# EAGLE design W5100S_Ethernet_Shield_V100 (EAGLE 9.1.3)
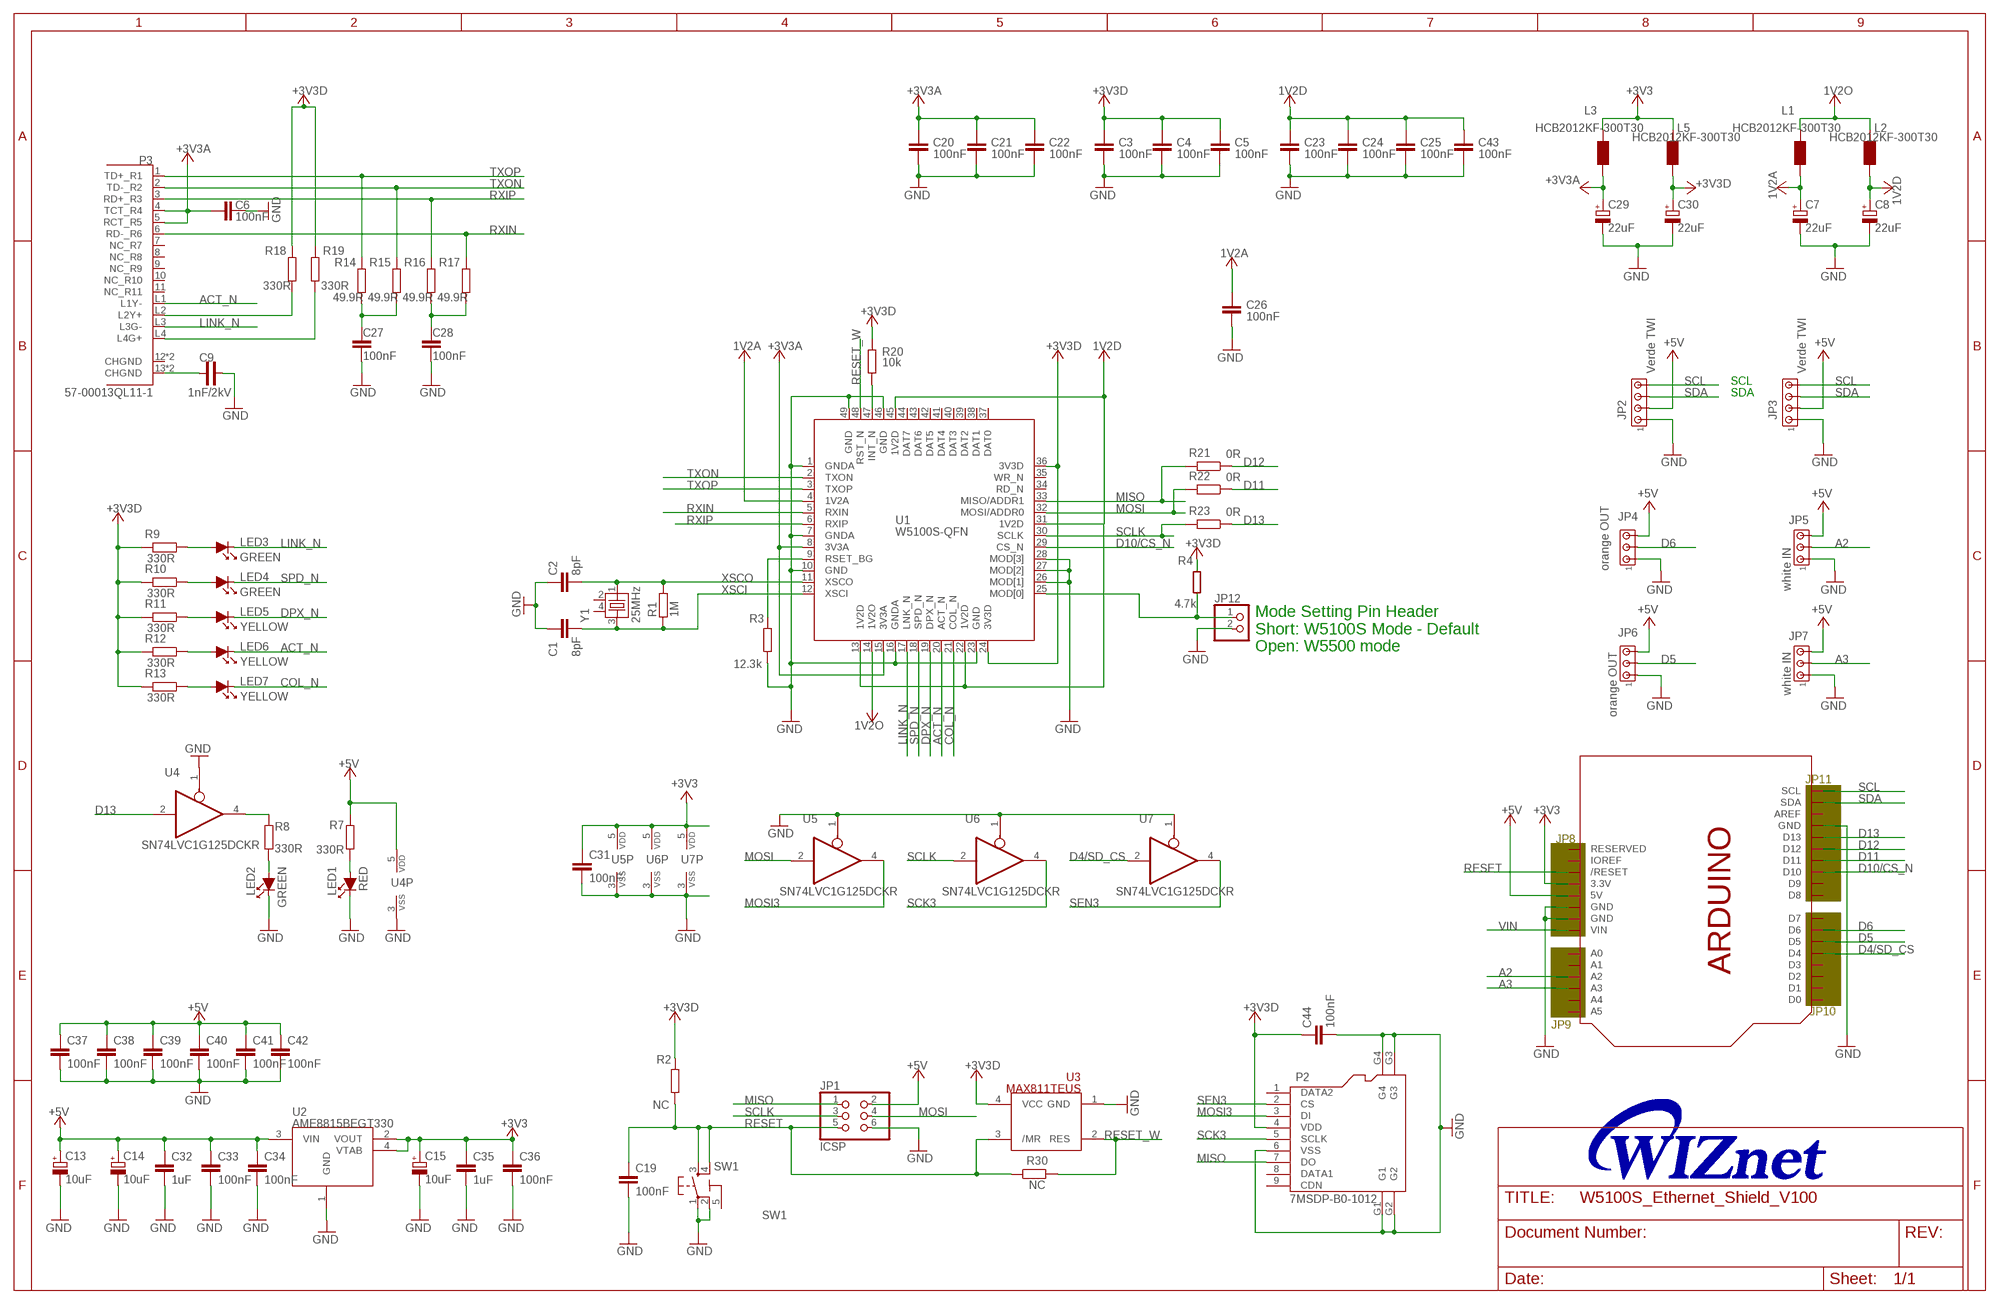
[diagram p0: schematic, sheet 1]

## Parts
C1  8pF  C-EU0603-RND  [C0603-ROUND]
C2  8pF  C-EU0603-RND  [C0603-ROUND]
C3  100nF  C-EU0603-RND  [C0603-ROUND]
C4  100nF  C-EU0603-RND  [C0603-ROUND]
C5  100nF  C-EU0603-RND  [C0603-ROUND]
C6  100nF  0142_10NF_0603  [C0603-ROUND@1]
C7  22uF  0474_TAJA475M016RNJ  [SMC_A]
C8  22uF  0474_TAJA475M016RNJ  [SMC_A]
C9  1nF/2kV  C-4520  [C-4520]
C13  10uF  0474_TAJA475M016RNJ  [SMC_A]
C14  10uF  0474_TAJA475M016RNJ  [SMC_A]
C15  10uF  0474_TAJA475M016RNJ  [SMC_A]
C19  100nF  0142_10NF_0603  [C0603-ROUND@1]
C20  100nF  C-EU0603-RND  [C0603-ROUND]
C21  100nF  C-EU0603-RND  [C0603-ROUND]
C22  100nF  C-EU0603-RND  [C0603-ROUND]
C23  100nF  C-EU0603-RND  [C0603-ROUND]
C24  100nF  C-EU0603-RND  [C0603-ROUND]
C25  100nF  C-EU0603-RND  [C0603-ROUND]
C26  100nF  C-EU0603-RND  [C0603-ROUND]
C27  100nF  0142_10NF_0603  [C0603-ROUND@1]
C28  100nF  0142_10NF_0603  [C0603-ROUND@1]
C29  22uF  0474_TAJA475M016RNJ  [SMC_A]
C30  22uF  0474_TAJA475M016RNJ  [SMC_A]
C31  100nF  0006_1UF_0603/GRM188R61E105KA12D  [C0603-ROUND]
C32  1uF  0142_10NF_0603  [C0603-ROUND@1]
C33  100nF  0142_10NF_0603  [C0603-ROUND@1]
C34  100nF  0142_10NF_0603  [C0603-ROUND@1]
C35  1uF  0142_10NF_0603  [C0603-ROUND@1]
C36  100nF  0142_10NF_0603  [C0603-ROUND@1]
C37  100nF  0142_10NF_0603  [C0603-ROUND@1]
C38  100nF  0142_10NF_0603  [C0603-ROUND@1]
C39  100nF  0142_10NF_0603  [C0603-ROUND@1]
C40  100nF  0142_10NF_0603  [C0603-ROUND@1]
C41  100nF  0142_10NF_0603  [C0603-ROUND@1]
C42  100nF  0142_10NF_0603  [C0603-ROUND@1]
C43  100nF  C-EU0603-RND  [C0603-ROUND]
C44  100nF  0006_1UF_0603/GRM188R61E105KA12D  [C0603-ROUND]
JP1  ICSP  0114_PH254-203DF118A00V  [2X03]
JP2  Verde TWI  1693_WA254-04S-632  [10X04MTA]
JP3  Verde TWI  1693_WA254-04S-632  [10X04MTA]
JP4  orange OUT  1696_WA254-03S-166  [10X03MTA]
JP5  white IN  1695_WA254-03S-IN  [10X03MTA]
JP6  orange OUT  0141_LHA-03-TS  [10X03MTA]
JP7  white IN  1695_WA254-03S-IN  [10X03MTA]
JP12  PINHD-1X2  [1X02]
L1  HCB2012KF-300T30  0001_BLM21PG300SN1D_/_MH2029-300Y  [0805]
L2  HCB2012KF-300T30  0001_BLM21PG300SN1D_/_MH2029-300Y  [0805]
L3  HCB2012KF-300T30  0001_BLM21PG300SN1D_/_MH2029-300Y  [0805]
L5  HCB2012KF-300T30  0001_BLM21PG300SN1D_/_MH2029-300Y  [0805]
LED1  RED  LED-1608  [LED-1608]
LED2  GREEN  LED-1608  [LED-1608]
LED3  GREEN  LED-1608  [LED-1608]
LED4  GREEN  LED-1608  [LED-1608]
LED5  YELLOW  LED-1608  [LED-1608]
LED6  YELLOW  LED-1608  [LED-1608]
LED7  YELLOW  LED-1608  [LED-1608]
P2  7MSDP-B0-1012  MICRO-SD-CARD-SOCKET-9P(ST-TF-003A)  [MICRO-SD9+4P-SMD-16.1X14.5X1.85MM]
P3  57-00013QL11-1  [57-00013QL11-1]
R1  1M  RESISTENZE_0026_100K_0603  [RESISTENZE_R0603-ROUND]
R2  NC  0028_CR0603JW103L  [R0603-ROUND]
R3  12.3k  0028_CR0603JW103L  [R0603-ROUND]
R4  4.7k  R-330R-0402  [0402-1005X55N]
R7  330R  RESISTENZE_0026_100K_0603  [RESISTENZE_R0603-ROUND]
R8  330R  RESISTENZE_0026_100K_0603  [RESISTENZE_R0603-ROUND]
R9  330R  0028_CR0603JW103L  [R0603-ROUND]
R10  330R  0028_CR0603JW103L  [R0603-ROUND]
R11  330R  0028_CR0603JW103L  [R0603-ROUND]
R12  330R  0028_CR0603JW103L  [R0603-ROUND]
R13  330R  0028_CR0603JW103L  [R0603-ROUND]
R14  49.9R  RESISTENZE_0026_100K_0603  [RESISTENZE_R0603-ROUND]
R15  49.9R  RESISTENZE_0026_100K_0603  [RESISTENZE_R0603-ROUND]
R16  49.9R  RESISTENZE_0026_100K_0603  [RESISTENZE_R0603-ROUND]
R17  49.9R  RESISTENZE_0026_100K_0603  [RESISTENZE_R0603-ROUND]
R18  330R  RESISTENZE_0026_100K_0603  [RESISTENZE_R0603-ROUND]
R19  330R  RESISTENZE_0026_100K_0603  [RESISTENZE_R0603-ROUND]
R20  10k  0028_CR0603JW103L  [R0603-ROUND]
R21  0R  0028_CR0603JW103L  [R0603-ROUND]
R22  0R  0028_CR0603JW103L  [R0603-ROUND]
R23  0R  0028_CR0603JW103L  [R0603-ROUND]
R30  NC  0028_CR0603JW103L  [R0603-ROUND]
SW1  SW1  0946_TS42031-160W-TR-7260  [TS42]
U1  W5100S-QFN  [W5100S-QFN]
U2  AME8815BEGT330  [SOT-223]
U3  MAX811TEUS  0035_CAT811TTBI-GT3  [SOT143]
U4  SN74LVC1G125DCKR  0040_SN74LVC1G125DCKR  [SC70-5]
U5  SN74LVC1G125DCKR  0040_SN74LVC1G125DCKR  [SC70-5]
U6  SN74LVC1G125DCKR  0040_SN74LVC1G125DCKR  [SC70-5]
U7  SN74LVC1G125DCKR  0040_SN74LVC1G125DCKR  [SC70-5]
U$4  ARDUINO_R3_ICSP_4  [ARDUINOR3_ICSP_4]
Y1  25MHz  XTAL3225  [XTAL3225]

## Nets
1V2A: C7.+ C26.2 L1.1 U1.4(1V2A)
1V2D: C8.+ C23.2 C24.2 C25.2 C43.2 L2.1 U1.13(1V2D) U1.22(1V2D) U1.31(1V2D) U1.45(1V2D)
1V2O: L1.2 L2.2 U1.14(1V2O)
+3V3 [power]: C15.+ C31.1 C35.1 C36.1 L3.2 L5.2 U2.2(VOUT) U2.4(VTAB) U5.5(VDD) U6.5(VDD) U7.5(VDD) U$4.3V(3.3V)
+3V3A [power]: C6.1 C20.2 C21.2 C22.2 C29.+ L3.1 P3.4(TCT_R4) P3.5(RCT_R5) U1.8(3V3A) U1.15(3V3A)
+3V3D: C3.2 C4.2 C5.2 C30.+ C44.1 L5.1 P2.4(VDD) R2.2 R4.2 R9.2 R10.2 R11.2 R12.2 R13.2 R18.1 R19.1 R20.2 U1.24(3V3D) U1.36(3V3D) U3.4(VCC)
+5V [power]: C13.+ C14.+ C32.1 C33.1 C34.1 C37.1 C38.1 C39.1 C40.1 C41.1 C42.1 JP1.2 JP2.2 JP3.2 JP4.3 JP5.3 JP6.3 JP7.3 R7.2 U2.3(VIN) U4.5(VDD) U$4.5V
A2: JP5.2 U$4.A2
A3: JP7.2 U$4.A3
ACT_N: LED6.K P3.L1(L1Y-) U1.20(ACT_N)
COL_N: LED7.K U1.21(COL_N)
D4/SD_CS: U7.2(I) U$4.D4
D5: JP6.2 U$4.D5
D6: JP4.2 U$4.D6
D10/CS_N: U1.29(CS_N) U$4.D10
D11: R22.1 U$4.D11
D12: R21.1 U$4.D12
D13: R23.1 U4.2(I) U$4.D13
DPX_N: LED5.K U1.19(DPX_N)
GND [gnd]: C1.1 C2.1 C3.1 C4.1 C5.1 C6.2 C7.- C8.- C9.2 C13.- C14.- C15.- C19.2 C20.1 C21.1 C22.1 C23.1 C24.1 C25.1 C26.1 C27.1 C28.1 C29.- C30.- C31.2 C32.2 C33.2 C34.2 C35.2 C36.2 C37.2 C38.2 C39.2 C40.2 C41.2 C42.2 C43.1 C44.2 JP1.6 JP2.1 JP3.1 JP4.1 JP5.1 JP6.1 JP7.1 JP12.2 LED1.K LED2.K P2.6(VSS) P2.G1 P2.G2 P2.G3 P2.G4 R3.1 SW1.1 SW1.2 U1.1(GNDA) U1.7(GNDA) U1.10(GND) U1.16(GNDA) U1.23(GND) U1.26(MOD[1]) U1.27(MOD[2]) U1.28(MOD[3]) U1.46(GND) U1.49(GND) U2.1(GND) U3.1(GND) U4.1(OE) U4.3(VSS) U5.1(OE) U5.3(VSS) U6.1(OE) U6.3(VSS) U7.1(OE) U7.3(VSS) U$4.GND U$4.GND@1(GND) U$4.GND@2(GND)
LINK_N: LED3.K P3.L3(L3G-) U1.17(LNK_N)
MISO: JP1.1 P2.7(DO) R21.2 U1.33(MISO/ADDR1)
MOSI: JP1.4 R22.2 U1.32(MOSI/ADDR0) U5.2(I)
MOSI3: P2.3(DI) U5.4(O)
N$1: LED3.A R9.1
N$2: P3.L2(L2Y+) R18.2
N$3: LED1.A R7.1
N$4: LED4.A R10.1
N$5: LED5.A R11.1
N$6: LED6.A R12.1
N$7: LED7.A R13.1
N$8: P3.L4(L4G+) R19.2
N$9: C9.1 P3.13(CHGND) P3.P$4(CHGND)
N$12: C27.2 R14.2 R15.2
N$13: R8.2 U4.4(O)
N$14: LED2.A R8.1
N$15: C28.2 R16.2 R17.2
N$16: R20.1 U1.47(INT_N)
N$17: JP12.1 R4.1 U1.25(MOD[0])
N$20: R3.2 U1.9(RSET_BG)
RESET: C19.1 JP1.5 R2.1 R30.1 SW1.3 SW1.4 U3.3(/MR) U$4.RESET(/RESET)
RESET_W: R30.2 U1.48(RST_N) U3.2(RES)
RXIN: P3.6(RD-_R6) R17.1 U1.5(RXIN)
RXIP: P3.3(RD+_R3) R16.1 U1.6(RXIP)
SCK3: P2.5(SCLK) U6.4(O)
SCL: JP2.4 JP3.4 U$4.SCL
SCLK: JP1.3 R23.2 U1.30(SCLK) U6.2(I)
SDA: JP2.3 JP3.3 U$4.SDA
SEN3: P2.2(CS) U7.4(O)
SPD_N: LED4.K U1.18(SPD_N)
TXON: P3.2(TD-_R2) R15.1 U1.2(TXON)
TXOP: P3.1(TD+_R1) R14.1 U1.3(TXOP)
VIN [gnd]: U$4.VIN
XSCI: C1.2 R1.1 U1.12(XSCI) Y1.3
XSCO: C2.2 R1.2 U1.11(XSCO) Y1.1
Unconnected: P2.1(DATA2) P2.8(DATA1) P2.9(CDN) P3.7(NC_R7) P3.8(NC_R8) P3.9(NC_R9) P3.10(NC_R10) P3.11(NC_R11) P3.12(CHGND) P3.P$3(CHGND) U1.34(RD_N) U1.35(WR_N) U1.37(DAT0) U1.38(DAT1) U1.39(DAT2) U1.40(DAT3) U1.41(DAT4) U1.42(DAT5) U1.43(DAT6) U1.44(DAT7) U$4.A0 U$4.A1 U$4.A4 U$4.A5 U$4.AREF U$4.D0 U$4.D1 U$4.D2 U$4.D3 U$4.D7 U$4.D8 U$4.D9 U$4.IOREF U$4.RESERVED Y1.2 Y1.4

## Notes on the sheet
- SCL
- SDA
- Mode Setting Pin Header
  Short: W5100S Mode - Default
  Open: W5500 mode
- JP11
- JP8
- JP10
- JP9

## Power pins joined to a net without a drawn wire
5-GND: SW1.5(5-GND)

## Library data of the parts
C1-C5 C20-C26 C43 = SmartPrj:C-EU: CAPACITOR, European symbol
C6 C19 C27 C28 C32-C42 = Condensatori:0142_10NF_0603: 10nF 0603; CASE: 0603; MONTHLY_USAGE: _____; PART_NUMBER: 10nF_0603; PRICE: _____; SUPPLIER: _____; TYPE: Condensatori; VALUE: 10nF
C7 C8 C13-C15 C29 C30 = Condensatori:0474_TAJA475M016RNJ: 4u7 tantalio Case A - testa gialla -Tantalio; CASE: CaseA_(1206); MONTHLY_USAGE: _____; PART_NUMBER: TAJA475M016RNJ; PRICE: _____; SUPPLIER: _____; TYPE: Condensatori; VALUE: 4u7
C9 = CAP:C-4520
C31 C44 = Condensatori:0006_1UF_0603/GRM188R61E105KA12D: 1uF 0603; CASE: 0603; MONTHLY_USAGE: 207014.16; PART_NUMBER: 1uF_0603/GRM188R61E105KA12D; PRICE: �_0.00; SUPPLIER: La_Tecnika_Due_s.r.l.; TYPE: Condensatori; VALUE: 1uF
JP1 = Connettori:0114_PH254-203DF118A00V: 3x2 M V h 8,5 mm p2,54; MONTHLY_USAGE: _____; PART_NUMBER: PH254-203DF118A00V; PRICE: _____; SUPPLIER: _____; TYPE: Connettori
JP2 JP3 = Connettori:1693_WA254-04S-632: 4x1 V Verde p 2,54 Serigrafato TWI; MONTHLY_USAGE: _____; PART_NUMBER: WA254-04S-632; PRICE: _____; SUPPLIER: _____; TYPE: Connettori; VALUE: WA254-04S-632
JP4 = Connettori:1696_WA254-03S-166: 3x1 Poli V Arancioni Serigrafati OUT; MONTHLY_USAGE: _____; PART_NUMBER: WA254-03S-166; PRICE: _____; SUPPLIER: _____; TYPE: Connettori; VALUE: WA254-03S-166
JP5 JP7 = Connettori:1695_WA254-03S-IN: 3x1 V Bianco P2,54 Serigrafati IN; MONTHLY_USAGE: _____; PART_NUMBER: WA254-03S-IN; PRICE: _____; SUPPLIER: _____; TYPE: Connettori; VALUE: WA254-03S-IN
JP6 = Connettori:0141_LHA-03-TS: 3x1 V Bianco P2,54; MONTHLY_USAGE: _____; PART_NUMBER: LHA-03-TS; PRICE: _____; SUPPLIER: _____; TYPE: Connettori; VALUE: LHA-03-TS
JP12 = PinHeader:PINHD-1X2: PIN HEADER
L1-L3 L5 = Protezione:0001_BLM21PG300SN1D_/_MH2029-300Y: BLM21; MONTHLY_USAGE: _____; PART_NUMBER: BLM21PG300SN1D_/_MH2029-300Y; PRICE: _____; SUPPLIER: _____; TYPE: Protezione; VALUE: MH2029-300Y
LED1-LED7 = DIODE:LED-1608
P2 = Seeed-OPL-Connector:MICRO-SD-CARD-SOCKET-9P(ST-TF-003A): 320090000; MPN: ST-TF-003A; VALUE: ST-TF-003A
P3 = WIZnet:57-00013QL11-1
R1 R7 R8 R14-R19 = Arduino-M0-V1:RESISTENZE_0026_100K_0603: 100K 0603; CASE: 0603; MONTHLY_USAGE: _____; PART_NUMBER: 100K_0603; PRICE: _____; SUPPLIER: _____; TYPE: Resistenze; VALUE: 100k
R2 R3 R9-R13 R21-R23 R30 = Resistenze:0028_CR0603JW103L: 10K 0603; CASE: 0603; MONTHLY_USAGE: _____; PART_NUMBER: CR0603JW103L; PRICE: _____; SUPPLIER: _____; TYPE: Resistenze; VALUE: 10k
R4 = MK1_Zero:R: Resistor; DESCR: RES 330 OHM 1/16W 1% 0402 SMD; MF: Yageo; MPN: RC0402FR-07330RL
R20 = Resistenze:0028_CR0603JW103L: 10K 0603; CASE: 0603; MONTHLY_USAGE: _____; PART_NUMBER: CR0603JW103L; PRICE: _____; SUPPLIER: _____; TYPE: Resistenze
SW1 = Switches:0946_TS42031-160W-TR-7260: Pushbutton 6x6 Smd - White; MONTHLY_USAGE: _____; PART_NUMBER: IT-1157AHNP-160G-G_GTR; PRICE: _____; SUPPLIER: _____; TYPE: Switches; VALUE: TS42
U1 = WIZnet:W5100S-QFN
U2 = RECULATOR:AME8815BEGT330
U3 = Circuito Integrato:0035_CAT811TTBI-GT3: 4-Pin Microprocessor Power Supply Supervisors- Reset Controller CAT811TTBI-GT3; CASE: SOT143-4; MONTHLY_USAGE: _____; PART_NUMBER: CAT811TTBI-GT3; PRICE: _____; SUPPLIER: _____; TYPE: Circuito_Integrato; VALUE: CAT811TTBI-GT3
U4-U7 = Circuito Integrato:0040_SN74LVC1G125DCKR: Single bus buffer with 3-state output; CASE: SC70; MONTHLY_USAGE: _____; PART_NUMBER: SN74LVC1G125DCKR; PRICE: _____; SPICEPREFIX: U; SUPPLIER: _____; TYPE: Circuito_Integrato; VALUE: 74LVC1G125DCKR
U$4 = Arduino:ARDUINO_R3_ICSP_4
Y1 = X-TAL:XTAL3225

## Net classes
1 power: width 0.254 mm, drill 0.61 mm, clearance 0.203 mm
2 gnd: width 0.254 mm, drill 0.3 mm, clearance 0.127 mm

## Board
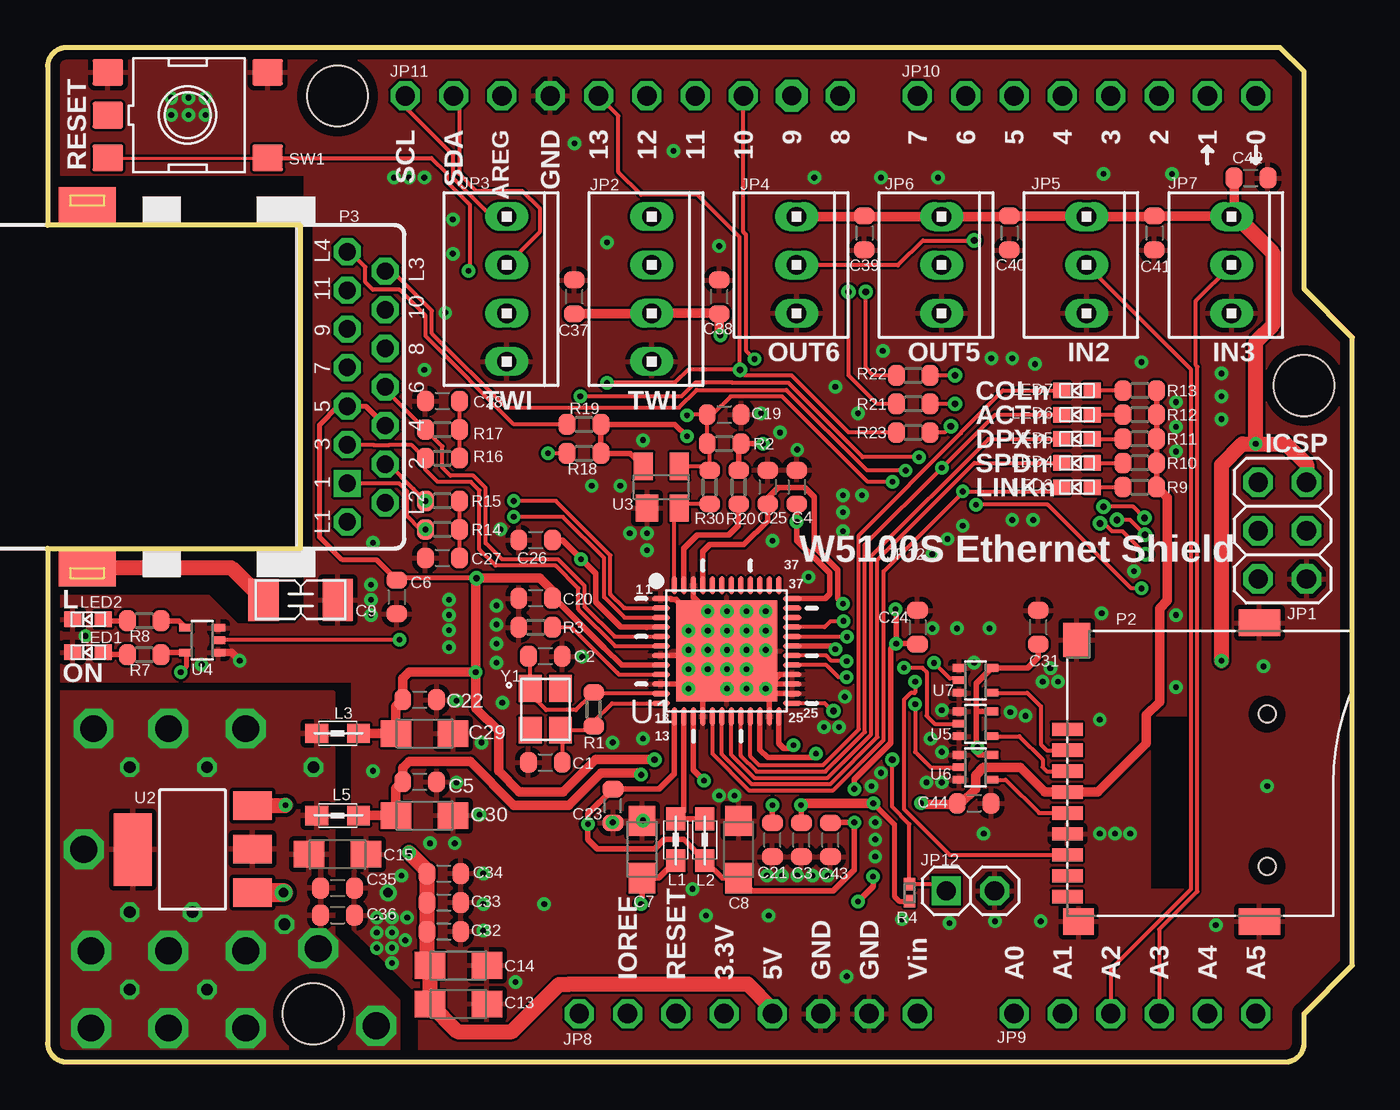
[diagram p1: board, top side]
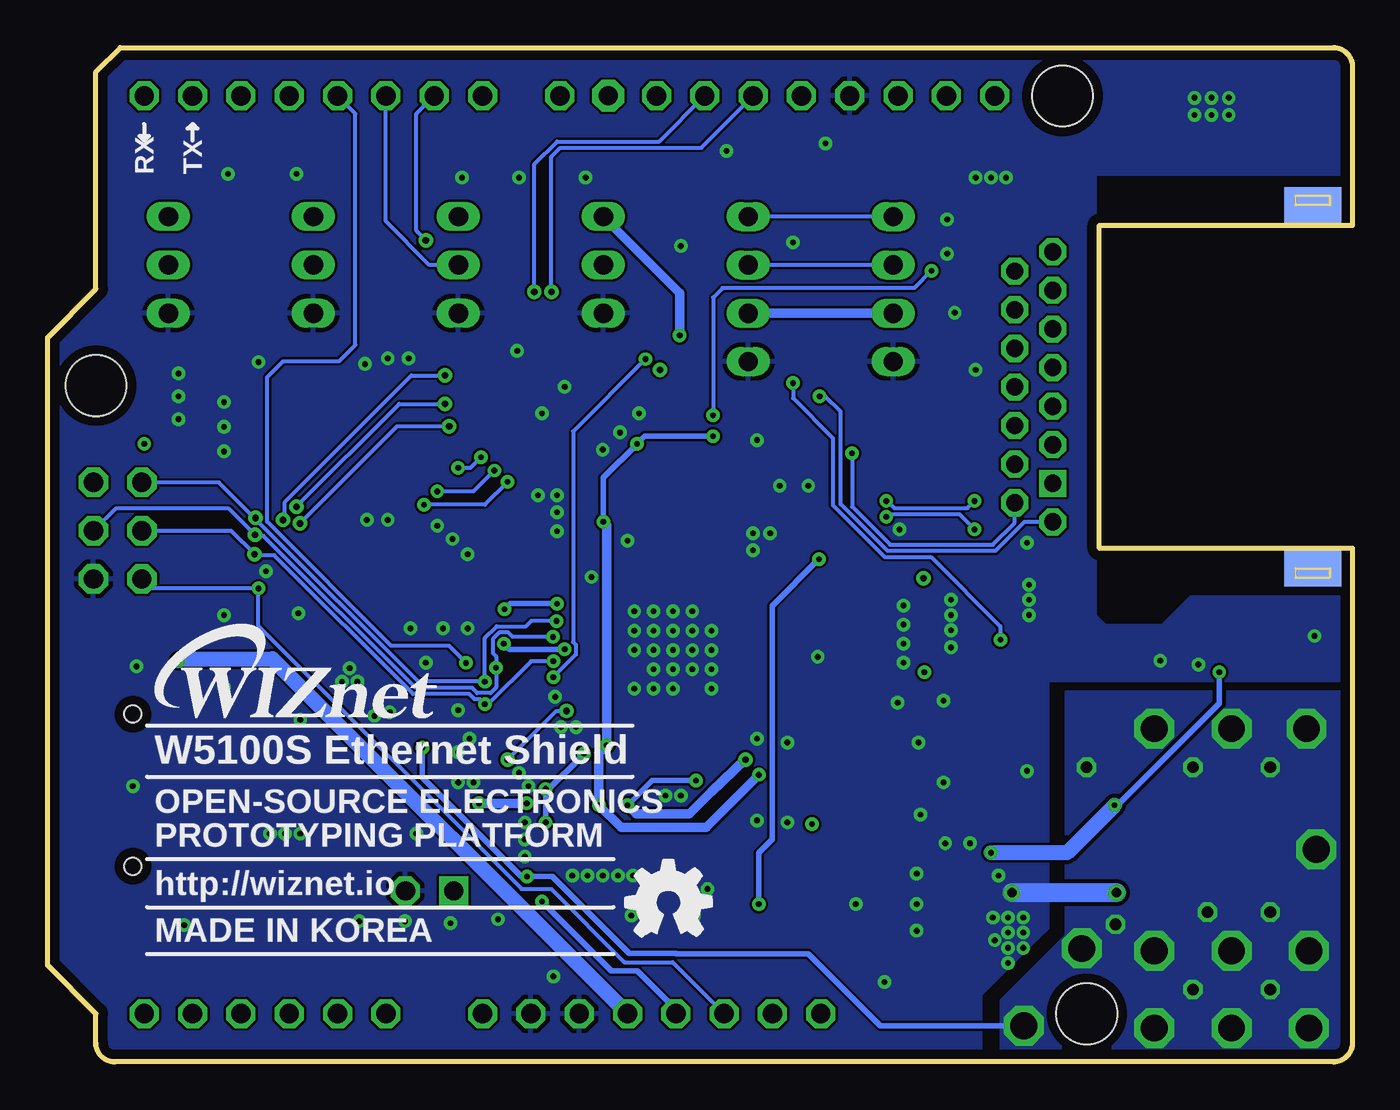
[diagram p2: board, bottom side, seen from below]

Size 68.58 x 53.34 mm. Coordinates in mm from the lower left corner, seen from the top.
Outline: 66.04,2.54 68.58,5.08 68.58,38.1 66.04,40.64 66.04,52.07 64.77,53.34 1,53.34 arc90 0,52.34 0,44 13.3,44 13.3,27 0,27 0,1 arc90 1,0 65.04,0 arc90 66.04,1 66.04,2.54
Copper layers (1*16): Top 0.035mm / dielectric 1.5mm / Bottom 0.035mm
Design rules "default *": minimum track width 6mil, minimum drill 0.2mm, track to track 5mil, track to pad 5mil, pad to pad 5mil, via to via 5mil, smd to smd 4mil, copper to edge 20mil, drill to drill 10mil, minimum pad ring 10mil, minimum via ring 8mil, stop-mask expansion 1mil, vias tented up to drill 15mil, thermal gap 10mil

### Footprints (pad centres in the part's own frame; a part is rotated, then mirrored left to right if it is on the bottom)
C0603-ROUND = smd 0.898 x 1.1: 1 -0.889,0; 2 0.889,0
C0603-ROUND@1 = smd 0.898 x 1.1: 1 -0.889,0; 2 0.889,0
SMC_A = smd 1.6 x 1.4: + -1.5,0; - 1.5,0
C-4520 = smd 1.6 x 2.2: 1 -1.95,0; 2 1.95,0
2X03 = drill 1.016 pad 1.55 octagon: 1 -2.54,-1.27; 2 -2.54,1.27; 3 0,-1.27; 4 0,1.27; 5 2.54,-1.27; 6 2.54,1.27
10X04MTA = drill 1.016 long: 1 3.81,0; 2 1.27,0; 3 -1.27,0; 4 -3.81,0
10X03MTA = drill 1.016 long: 1 2.54,0; 2 0,0; 3 -2.54,0
1X02 = drill 1.016 square: 1 -1.27,0 | drill 1.016 octagon: 2 1.27,0
0805 = smd 1.2 x 1: 1 -1.1,0; 2 1.1,0
LED-1608 = smd 0.89 x 0.82: A -0.8,0; K 0.8,0
MICRO-SD9+4P-SMD-16.1X14.5X1.85MM = smd 1.6 x 0.7: 1 0,2.25; 2 0,1.15; 3 0,0.05; 4 0,-1.05; 5 0,-2.15; 6 0,-3.25; 7 0,-4.35; 8 0,-5.45; 9 0,-6.55 | smd 1.6 x 1.4: G1 0.6,-7.85 | smd 2.2 x 1.4: G2 10.1,-7.85; G3 10.1,7.85 | smd 1.4 x 1.8: G4 0.5,6.95 | hole 0.9: 10.5,-4.95; 10.5,3.05
57-00013QL11-1 = drill 0.914 square: 1 5.075,10.15 | drill 0.914 octagon: 2 4.065,12.15; 3 3.045,10.15; 4 2.035,12.15; 5 1.015,10.15; 6 0.005,12.15; 7 -1.015,10.15; 8 -2.025,12.15; 9 -3.045,10.15; 10 -4.055,12.15; 11 -5.075,10.15; L1 7.105,10.15; L2 6.095,12.15; L3 -6.085,12.15; L4 -7.105,10.15 | smd 2 x 3: 12 -9.5,-3.51; 13 9.5,-3.51 | smd 2 x 3 bottom: P$3 -9.5,-3.51; P$4 9.5,-3.51
RESISTENZE_R0603-ROUND = smd 0.898 x 1.1: 1 -0.889,0; 2 0.889,0
R0603-ROUND = smd 0.898 x 1.1: 1 -0.889,0; 2 0.889,0
0402-1005X55N = smd 0.62 x 0.62: 1 -0.45,0; 2 0.45,0
TS42 = smd 1.6 x 1.4: 1 -4.2,2.25; 2 4.2,2.25; 3 -4.2,-2.25; 4 4.2,-2.25; 5 -4.2,0
W5100S-QFN = smd 0.95 x 0.25: 1 -3.45,2.75; 2 -3.45,2.25; 3 -3.45,1.75; 4 -3.45,1.25; 5 -3.45,0.75; 6 -3.45,0.25; 7 -3.45,-0.25; 8 -3.45,-0.75; 9 -3.45,-1.25; 10 -3.45,-1.75; 11 -3.45,-2.25; 12 -3.45,-2.75; 25 3.45,-2.75; 26 3.45,-2.25; 27 3.45,-1.75; 28 3.45,-1.25; 29 3.45,-0.75; 30 3.45,-0.25; 31 3.45,0.25; 32 3.45,0.75; 33 3.45,1.25; 34 3.45,1.75; 35 3.45,2.25; 36 3.45,2.75 | smd 0.25 x 0.95: 13 -2.75,-3.45; 14 -2.25,-3.45; 15 -1.75,-3.45; 16 -1.25,-3.45; 17 -0.75,-3.45; 18 -0.25,-3.45; 19 0.25,-3.45; 20 0.75,-3.45; 21 1.25,-3.45; 22 1.75,-3.45; 23 2.25,-3.45; 24 2.75,-3.45; 37 2.75,3.45; 38 2.25,3.45; 39 1.75,3.45; 40 1.25,3.45; 41 0.75,3.45; 42 0.25,3.45; 43 -0.25,3.45; 44 -0.75,3.45; 45 -1.25,3.45; 46 -1.75,3.45; 47 -2.25,3.45; 48 -2.75,3.45 | smd 5.3 x 5.3: 49 0,0
SOT-223 = smd 1.499 x 2.007: 1 -2.261,-3.15; 2 0.025,-3.15; 3 2.311,-3.15 | smd 3.81 x 2.007: 4 0,3.15
SOT143 = smd 1.2 x 1.44: 1 -0.75,-1.1 | smd 1 x 1.44: 2 0.95,-1.1; 3 0.95,1.1; 4 -0.95,1.1
SC70-5 = smd 0.4 x 0.7: 1 -0.65,-0.85; 2 0,-0.85; 3 0.65,-0.85; 4 0.65,0.85; 5 -0.65,0.85
ARDUINOR3_ICSP_4 = drill 1.016 octagon: 3V 35.56,2.54; 5V 38.1,2.54; A0 50.8,2.54; A1 53.34,2.54; A2 55.88,2.54; A3 58.42,2.54; A4 60.96,2.54; A5 63.5,2.54; AREF 23.876,50.8; D0 63.5,50.8; D1 60.96,50.8; D2 58.42,50.8; D3 55.88,50.8; D4 53.34,50.8; D5 50.8,50.8; D6 48.26,50.8; D7 45.72,50.8; D8 41.656,50.8; D10 36.576,50.8; D11 34.036,50.8; D12 31.496,50.8; D13 28.956,50.8; GND 26.416,50.8; GND@1 43.18,2.54; GND@2 40.64,2.54; IOREF 30.48,2.54; RESERVED 27.94,2.54; RESET 33.02,2.54; SCL 18.796,50.8; SDA 21.336,50.8; VIN 45.72,2.54 | drill 1 pad 1.676 octagon: D9 39.116,50.8 | hole 3.2: 66.04,35.56; 15.24,50.8; 13.97,2.54
XTAL3225 = smd 1.4 x 1.2: 1 -1.1,-0.8; 2 1.1,-0.8; 3 1.1,0.8; 4 -1.1,0.8

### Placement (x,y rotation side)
C1  26.16,15.75 0 top
C2  26.16,21.34 180 top
C3  39.62,11.68 90 top
C4  39.37,30.23 270 top
C5  19.56,14.73 180 top
C6  18.35,24.45 270 top
C7  31.24,11.18 90 top
C8  36.32,11.18 90 top
C9  13.3,24.3 0 top
C13  21.59,3.05 0 top
C14  21.59,5.08 0 top
C15  15.24,10.92 0 top
C19  35.56,34.04 0 top
C20  25.65,24.38 0 top
C21  38.1,11.68 90 top
C22  19.56,19.05 180 top
C23  29.72,13.46 90 top
C24  45.72,22.86 270 top
C25  37.85,30.23 270 top
C26  25.65,27.44 0 top
C27  20.75,26.5 0 top
C28  20.75,34.75 0 top
C29  19.81,17.27 0 top
C30  19.81,12.95 0 top
C31  52.07,22.86 90 top
C32  20.83,6.86 0 top
C33  20.83,8.38 0 top
C34  20.83,9.91 0 top
C35  15.24,9.14 0 top
C36  15.24,7.72 0 top
C37  27.69,40.23 90 top
C38  35.31,40.23 90 top
C39  42.93,43.59 270 top
C40  50.55,43.59 270 top
C41  58.17,43.59 270 top
C42  63.25,46.48 0 top
C43  41.15,11.68 90 top
C44  48.7,13.6 0 top
JP1  64.9,27.94 270 top
JP2  31.75,40.64 270 top
JP3  24.13,40.64 270 top
JP4  39.37,41.91 270 top
JP5  54.61,41.91 270 top
JP6  46.99,41.91 270 top
JP7  62.23,41.91 270 top
JP12  48.5,9 0 top
L1  33.02,11.68 90 top
L2  34.54,11.68 90 top
L3  15.24,17.27 180 top
L5  15.24,12.95 180 top
LED1  2.13,21.54 180 top
LED2  2.13,23.28 180 top
LED3  54.1,30.23 180 top
LED4  54.1,31.5 180 top
LED5  54.1,32.77 180 top
LED6  54.1,34.04 180 top
LED7  54.1,35.31 180 top
P2  53.59,15.24 0 top
P3  5.6,35.5 270 top
R1  28.7,18.54 90 top
R2  35.56,32.51 0 top
R3  25.65,22.86 0 top
R4  45.3,8.9 270 top
R7  5.08,21.42 0 top
R8  5.08,23.2 0 top
R9  57.4,30.23 0 top
R10  57.4,31.5 0 top
R11  57.4,32.77 0 top
R12  57.4,34.04 0 top
R13  57.4,35.31 0 top
R14  20.75,28 0 top
R15  20.75,29.5 0 top
R16  20.75,31.75 0 top
R17  20.75,33.25 0 top
R18  28.19,32 180 top
R19  28.19,33.53 180 top
R20  36.32,30.23 90 top
R21  45.5,34.6 0 top
R22  45.5,36.1 0 top
R23  45.5,33.1 0 top
R30  34.8,30.23 270 top
SW1  7.37,49.78 0 top
U1  35.69,21.62 0 top
U2  7.62,11.18 90 top
U3  32.26,30.23 0 top
U4  8.13,22.18 90 top
U5  48.77,17.78 270 top
U6  48.77,15.49 270 top
U7  48.77,20.07 270 top
U$3  [WIZNET2-LOGO]  63.85,16.91 0 bottom
U$4  0,0 0 top
U$5  [OSHP-LOGO]  39,6 0 bottom
Y1  26.16,18.54 270 top

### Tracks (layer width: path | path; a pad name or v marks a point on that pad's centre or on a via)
1V2A  (via drill 0.3)
  Top 0.3: L1.1 32.11,9.68 C7.+ 31.24,8.34 v31.2,8.3 | 31.48,22.86 31.11,22.86 | v28.04,26.44 27.94,26.54 | v28.04,26.44 28.8,25.68 28.8,24.2 30.14,22.86 31.48,22.86 | v28.04,26.44 27.04,27.44 C26.2 | 31.48,22.86 U1.4
  Bottom 0.3: v28.04,26.44 30.5,23.98 30.5,11.7 31.2,11 v31.2,8.3 31.2,8.2
1V2D  (via drill 0.3)
  Top 0.3: C8.+ 35.45,9.68 L2.1 33.43,11.7 32.4,11.7 31.9,11.2 28.9,11.2 28.4,11.7 v28.4,12.5 28.4,13.03 C23.2 32.15,14.35 32.94,15.14 U1.13 | 41.23,21.86 v41.4,21.7 41.23,21.86 | v44.6,22 45.69,22 C24.2 | v40.39,16.2 40.18,16 37.85,16 37.44,16.41 U1.22 | C43.2 41.17,12.6 v42.4,12.6 42.4,10.1 41.3,9 37,9 C8.+ | C8.+ 36.6,9.4 | v44.6,22 44.32,21.72 44.32,16.79 42.4,14.87 v42.4,14.36 | v44.6,22 44.6,23.76 v44.56,23.8 | v41.8,24.1 41.53,24.37 41.53,25.88 40.3,27.1 40.3,29.7 39.8,30.2 38.4,30.2 37.85,29.65 C25.2 37.85,28.45 36.6,27.2 34.8,27.2 34.44,26.84 U1.45 | 41.23,21.86 U1.31
  Bottom 0.3: v41.4,21.7 44.3,21.7 v44.6,22 | v40.39,16.2 42.4,14.19 | 42.4,14.19 v42.4,12.6 | v42.4,14.36 42.4,14.19 | v44.56,23.8 44.26,24.1 v41.8,24.1
1V2O
  Top 0.3: L2.2 L1.2 33.44,13.2 U1.14
+3V3  (via drill 0.3, 0.61, 1.4)
  Top 0.3: U6.5 48.96,16.14 48.8,16.3 48.8,16.46 | 48.8,16.46 48.8,18.5 | 48.8,18.5 48.8,19.9 U7.5 51.52,20.72 52.07,21.27 C31.1 | U5.5 48.87,18.43 48.8,18.5 | 48.8,16.46 v48.88,16.54 | v43.39,9.75 43.39,9.22 v42.6,8.44
  Bottom 0.254: U$4.3V 35.56,2.76
  Bottom 0.3: v48.88,16.54 48.88,14.95 43.67,9.75 v43.39,9.75 42.05,9.75 38.01,5.71 35.55,5.71 35.54,5.7 28.6,5.7 24.8,1.91 v17.27,1.91 | v42.6,8.44 38.96,4.8 37.6,4.8 35.56,2.76
  other vias: 4.32,7.87 7.62,7.87 6.35,5.84 10.41,5.84 4.32,3.81 8.38,3.81 2.29,5.84 6.35,1.78 10.41,1.78 2.29,1.78 12.45,7.24 14.22,5.97 1.91,11.18 1.91,11.18 2.41,17.53 6.35,17.53 4.32,15.49 8.38,15.49 13.97,15.49 10.41,17.53
  pour Top: 0,0 18.4,0 18.4,3.2 16.4,5.2 15,6.6 15,7 15,10.4 15,16.8 15,19.4 0,19.4
  pour Bottom: 0,-0.2 18.4,-0.2 18.4,3.2 15,6.6 15,19.4 0,19.4
+3V3A  (via drill 0.3, 0.35)
  Top 0.254: v22.54,25.44 18.45,25.44 C6.1 17.29,26.4 15.5,26.4 14.3,27.6 14.3,33.5 15.29,34.48 P3.5 16.73,34.48 P3.4
  Top 0.3: 29.26,21.78 | 29.26,21.78 30.18,20.86 U1.8 | v38.1,13.5 C21.2 | v34.5,14.8 33.94,15.36 U1.15 | C20.2 26.66,24.38 29.26,21.78
  Top 0.5: L3.1 C29.+ 18.31,18.69 C22.2 18.67,20.17 19,20.5 v22.5,20.5 | v22.5,20.5 22.5,18.6 23.7,17.4 23.7,15.3 24.8,14.2 27.1,14.2 28.81,15.91 31.53,15.91 31.54,15.9 v31.9,15.9 | v22.5,20.5 22.5,25.4 v22.54,25.44 25.87,25.44 26.54,24.77 C20.2
  Bottom 0.3: v34.5,14.8 36.8,14.8 v38.1,13.5
  Bottom 0.5: v31.9,15.9 33.7,14.2 34.86,13.04 37.64,13.04 v38.1,13.5
+3V3D  (via drill 0.3)
  Top 0.254: v43.4,13.6 44.5,12.5 44.5,8.7 44.75,8.45 R4.2
  Top 0.3: C4.2 v39.37,28.4 39.37,27.43 41.1,25.7 41.1,24.6 40.87,24.36 U1.36 | v39.6,13.5 39.6,12.6 C3.2 | R13.2 R12.2 R11.2 R10.2 R9.2 | R20.2 36.32,32.38 R2.2 37.59,32.51 v37.6,32.5 | v39.2,16.66 39.04,16.5 38.7,16.5 38.44,16.76 U1.24 | v33.6,32.9 32.97,33.53 R19.1 R18.1 30.63,32 U3.4
  Top 0.5: L5.1 C30.+ 18.31,14.38 C5.2 18.67,15.47 19,15.8 22.21,15.8 24.51,13.5 27.39,13.5 29.09,15.2 31.1,15.2 v31.2,15.1 | 39.64,13.54 v39.6,13.5 39.7,13.6 v43.4,13.6 | v45.9,13.6 45.96,13.54 47.75,13.54 C44.1 48.01,13.6 48.77,14.37 48.77,15.08 49.18,15.49 51.11,15.49 52.41,14.19 P2.4 55.19,14.19 57.74,16.74 57.74,18.24 58.44,18.94 58.44,23.86 58.84,24.26 58.84,29.68 R9.2
  Bottom 0.3: v39.37,28.4 39.37,30.73 v37.6,32.5 37.2,32.9 v33.6,32.9
  Bottom 0.5: v45.9,13.6 v43.4,13.6 | v39.37,28.4 39.2,28.23 v39.2,16.66 39.6,16.26 v39.6,13.5 38.44,12.34 33.96,12.34 v31.2,15.1
+5V  (via drill 0.3)
  Top 0.254: U4.5 7.28,20.78 v7,20.5 | U$4.5V 38.1,2.8
  Top 0.3: C14.+ | U4.5 6.08,21.53 R7.2
  Top 0.5: C34.1 | 27.66,39.37 C37.1 31.72,39.34 JP2.2 35.28,39.37 C38.1 35.31,38.25 v35.36,38.2 | C42.1 62.36,44.58 62.26,44.48 | 62.26,44.48 JP7.3 | JP4.3 42.9,44.45 C39.1 42.95,44.45 JP6.3 50.52,44.45 C40.1 54.58,44.48 JP5.3 58.14,44.45 C41.1 62.26,44.48
  Top 0.8: U2.3 12.49,13.49 v12.5,13.5 | v19,11 19.93,10.07 C34.1 | C34.1 C33.1 C32.1 19.94,5.23 C14.+ | C14.+ C13.+ 21.54,1.6 24.4,1.6 26.88,4.08 27.39,4.08 27.41,4.1 36.8,4.1 38.1,2.8 | v61.7,21.1 61.7,31.4 62.8,32.5 v63.5,32.5 | v63.5,32.5 65.1,32.5 66.17,31.43 JP1.2 | v63.5,32.5 63.5,37.88 64.41,38.78 64.41,42.53 62.36,44.58
  Bottom 0.3: v12.5,13.5 12.36,13.5 7,18.86 v7,20.5
  Bottom 0.5: JP3.2 JP2.2 | v35.36,38.2 35.36,40.44 JP4.3
  Bottom 0.8: v12.5,13.5 15,11 v19,11 | v61.7,21.1 61.4,21.2 56.76,21.2 U$4.5V
A2
  Top 0.2: JP5.2 60.1,36.42 60.1,9.11 55.88,4.88 U$4.A2
A3
  Top 0.2: JP7.2 60.35,40.03 60.35,36.63 60.43,36.55 60.43,8.97 58.42,6.96 U$4.A3
ACT_N  (via drill 0.3)
  Top 0.2: LED6.K 49.8,34.04 v47,31.24 42.96,27.2 42.96,17.35 40.88,15.27 37.27,15.27 36.44,16.1 U1.20 | v45.8,31.8 42.83,31.8 38.92,35.72 36,35.72 | v28,35 33.32,35 34.03,35.71 34.03,35.72
  Top 0.203: 36,35.72 34.03,35.72
  Bottom 0.2: v45.8,31.8 46.36,31.24 v47,31.24 | P3.L1 17.24,28.39 18.77,26.87 24.43,26.87 26.9,29.34 26.9,34.2 27.7,35 v28,35
COL_N
  Top 0.2: LED7.K 50.21,35.31 48,33.1 48,33.06 42.63,27.69 42.63,17.49 40.75,15.6 37.4,15.6 36.94,16.06 U1.21
D4/SD_CS  (via drill 0.3)
  Top 0.2: U7.2 47.82,20.16 47.42,20.16 46.6,20.98 v46.58,20.98
  Bottom 0.2: v46.58,20.98 47.5,21.9 50.54,21.9 57.05,28.41 57.05,36.01 56.2,36.85 53.25,36.85 52.4,37.7 52.4,49.86 U$4.D4
D5
  Bottom 0.2: JP6.2 48.51,41.91 50.8,44.2 U$4.D5
D6  (via drill 0.35)
  Top 0.2: v48.7,43.2 46,43.2 44.7,41.9 39.38,41.9 JP4.2
  Bottom 0.2: v48.7,43.2 49.2,43.7 49.2,49.86 U$4.D6
D10/CS_N  (via drill 0.3)
  Top 0.2: v42,20.24 41.56,20.24 40.94,20.86 U1.29 | v37.16,36.96 36.7,37.41 36.7,43.51 36.58,43.64 U$4.D10
  Bottom 0.2: v42,20.24 40.82,21.42 40.82,21.94 40.96,22.08 40.96,33.16 v37.16,36.96
D11  (via drill 0.35)
  Top 0.2: R22.1 43.4,36.1 43,36.5 v43,40.5
  Bottom 0.2: v43,40.5 43,47.2 41.8,48.4 36.44,48.4 U$4.D11
D12  (via drill 0.35)
  Top 0.2: R21.1 43.6,34.6 42.1,36.1 v42.1,40.5
  Bottom 0.2: v42.1,40.5 42.1,47.6 41.63,48.07 34.22,48.07 U$4.D12
D13  (via drill 0.3, 0.35)
  Top 0.2: U4.2 8.96,22.2 8.8,22.2 18.3,22.2 v18.5,22.2 | 36.38,36.42 36.38,36.5 | 36.38,36.5 36.38,43.38 34.16,45.6 31.2,45.6 30,46.8 30,49.76 U$4.D13 | R23.1 42.1,33.1 39.1,36.1 36.66,36.1 36.43,36.33 | 36.43,36.33 36.38,36.38 36.38,36.5 | v29.4,35.7 29.41,35.71 32.97,35.71 33.66,36.4 v36.4,36.4 36.4,36.36 36.43,36.33
  Bottom 0.2: v29.4,35.7 29.4,34.9 27.3,32.8 27.3,29.27 24.57,26.55 22.15,26.55 18.5,22.9 v18.5,22.2
DPX_N
  Top 0.2: LED5.K 49.45,32.77 43.29,26.6 43.29,17.22 41.02,14.95 37.13,14.95 35.94,16.14 U1.19
GND  (via drill 0.3, 0.5)
  Top 0.3: U1.16 34.44,20.39 v34.7,20.65 | 33.22,19.88 33.47,19.63 v33.68,19.63 33.44,19.87 U1.10 | U1.23 37.94,19.24 | 37.94,19.24 37.94,19.44 v37.75,19.63 37.85,19.74 | U1.26 38.06,19.36 37.94,19.24 | U1.28 38.48,20.36 37.85,19.74 | U1.27 37.98,19.86 37.85,19.74 | U1.46 33.94,24.46 v34.7,23.7 34.42,23.42 33.91,23.42 33.01,24.31 32.77,24.31 32.72,24.36 U1.1 | U1.7 33.38,21.36 v33.68,21.66
  Top 0.406: U4.1 9.67,21.53 v10.1,21.1
  Top 1: U2.1 12.38,8.91 v12.4,8.9
  Bottom 1: v12.4,8.9 v17.9,8.9
  other vias: 41.8,27.9 28.1,21.3 35.3,14 29.7,12.6 37.8,9.8 38.6,9.8 39.4,9.8 40.2,9.8 41,9.8 36.1,14 48.7,21 47,18.5 47,16.3 47,14.7 46.4,17 46.2,14.7 43.3,14.5 43.8,15.2 43.5,12.6 43.5,11.7 43.5,10.8 47.4,7.3 49.2,12 44.9,7.5 42,4.5 46.5,22.8 47.8,22.8 52.3,20 55.4,23.6 59.3,23.5 59.3,19.7 55.3,18 17.3,7.6 18.1,7.6 18.9,7.6 18.1,5.2 18.1,6.8 17.3,6.8 17.3,6 18.1,6 18.8,6.4 18.6,9.8 22.7,13 21.5,14.7 21.4,11.5 22.8,16.8 21.5,19 17.1,15.3 29.7,16.8 23.9,18.9 23.6,24 23.6,23 23.6,22 23.6,21 31.5,27.8 31.5,26.9 30.6,27.8 39.4,32.2 42.8,29.8 38.5,33.1 21.1,23.5 21.1,22.7 17,25.1 21.1,21.8 17,23.5 2,22.4 8.1,20.9 7.4,49.8 7.4,50.7 8.3,50.7 8.3,49.8 6.5,49.8 6.5,50.7 41.8,29.8 41.8,28.9 51.8,28.5 57.5,36.8 59.3,32.1 42.6,34.1 41.4,35.5 49.6,37 50.7,37 51.9,36.7 61.7,36.2 59.1,46.7 55.5,46.7 46.8,46.5 43.8,46.5 40.3,46.5 27.7,48.3 32.9,47.9 35.3,42.9 29.4,43.1 53.1,20 51.4,18.2 52.2,7.4 61.4,7.2 49.8,7.4 37.9,7.7 33.9,9.1 24.6,4.2 22.9,6.9 22.9,8.3 22.9,9.9 20.1,11.5 41.9,19.2 41.6,17.6 40.8,17.6 49.5,22.8 59.3,34.7 61.7,35 59.3,33.4 21.3,44.3 21.3,42.5 20.9,39.4 18.2,46.5 19,46.5 19.8,46.5 34.6,7.7 31.3,12.7 31.3,17 55.3,12 56.1,12 56.9,12 64.1,14.5 63.9,20.8 57.1,25.8 61.7,33.8 38.1,27.4 37.5,34.1 30.1,30.3 40,25.5 35.71,21.66 35.71,22.68 35.71,23.7 35.71,20.65 35.71,19.63 34.7,21.66 33.68,20.65 36.73,21.66 37.75,21.66 36.73,20.65 36.73,19.63 33.68,22.68 34.7,22.68 36.73,22.68 36.73,23.7 37.75,22.68 37.75,23.7 17,24.3 21.1,24.3 28.6,30.3 50.7,28.5 43.9,37.4 46.5,26.7 47.3,27.5 48.1,28.2 52.7,20.7 50.6,18.4 17.1,27.3 23.8,28 31.3,32.7 26.1,8.3 19.8,36.4
  pour Top: -0.5,24.5 -0.5,20 16,20 16,7 16.5,6.5 19.5,3.5 19.5,-0.5 69.5,-0.5 69.5,54 39.5,54 -0.5,54 -0.5,46.65 13.5,46.65 13.5,23.5 13,23 10,23 8.5,24.5
  pour Bottom: -1.5,24.5 -1.5,20 16,20 16,7 16.5,6.5 19.5,3.5 19.5,-1.5 70.5,-1.5 70.5,55 39,55 -1.5,55 -1.5,46.63 13.5,46.63 13.5,23.5 13,23 10,23 8.5,24.5
LINK_N  (via drill 0.3)
  Top 0.2: LED3.K 53.05,29.97 48.11,29.97 | 48.11,29.97 43.94,25.8 43.94,16.95 41.29,14.29 36.86,14.29 34.94,16.21 U1.17 | v45.1,31.1 43.07,31.1 38.84,35.34 34.11,35.34 33.18,34.4 24.1,34.4 20.19,38.31 20.19,39.5 18.11,41.59 P3.L3 | v48.1,30 48.11,29.99 48.11,29.97
  Bottom 0.2: v45.1,31.1 46.2,30 v48.1,30
MISO  (via drill 0.3, 0.35)
  Top 0.2: v41.84,23.18 41.16,23.18 40.84,22.86 U1.33 | P2.7 47.41,10.89 45,13.3 45,19.04 45.36,19.4 45.56,19.4 45.6,19.44 v45.6,20 | v57.65,28.61 57.05,29.2 v55.5,29.2 | v47.7,34.6 R21.2
  Bottom 0.2: v41.84,23.18 43.17,23.18 43.45,22.91 44.98,22.91 45.6,22.28 v45.6,20 49.1,20 57.5,28.4 | 57.5,28.4 59.58,30.48 JP1.1 | 57.5,28.4 57.5,28.45 v57.65,28.61 | v55.5,29.2 50.1,34.6 v47.7,34.6
MOSI  (via drill 0.3, 0.35)
  Top 0.2: v45,20.73 45.97,20.73 46.2,20.5 46.2,18.2 46.62,17.78 U5.2 | v56.2,28.5 56.9,28.5 57.05,28.36 | v57.68,27.72 57.4,28 57.05,28.36 | 57.05,28.36 | v47.7,36.1 R22.2 | U1.32 39.15,22.35 v42.01,22.35
  Bottom 0.2: v42.01,22.35 44.13,22.35 44.36,22.58 44.84,22.58 45.18,22.24 45.18,21.5 45,21.32 v45,20.73 45,19.7 45.3,19.4 46,19.4 46.27,19.67 49.23,19.67 57.23,27.67 57.62,27.67 v57.68,27.72 59.06,29.1 65.01,29.1 JP1.4 | v56.2,28.5 56.1,28.59 56.1,29.45 49.46,36.1 v47.7,36.1
MOSI3
  Top 0.2: U5.4 51.07,17.13 52.3,15.9 52.3,15.5 52.51,15.29 P2.3
N$1
  Top 0.2: LED3.A R9.1
N$2  (via drill 0.3)
  Top 0.2: 27.3,32.42 R18.2 v26.3,32
  Bottom 0.2: v26.3,32 26.3,29.2 24.3,27.2 18.9,27.2 17.75,28.35 P3.L2
N$3
  Top 0.3: R7.1 3.06,21.42 LED1.A
N$4
  Top 0.2: LED4.A R10.1
N$5
  Top 0.2: LED5.A R11.1
N$6
  Top 0.2: LED6.A R12.1
N$7
  Top 0.2: R13.1 LED7.A
N$8
  Top 0.2: R19.2 24.51,33.53 19.87,38.17 19.87,39.23 18.5,40.6 17.1,40.6 16.7,41 16.7,41.8 15.89,42.6 P3.L4
N$9
  Top 0.8: P3.P$4 9.65,26 C9.1
N$12
  Top 0.2: R15.2 R14.2 C27.2
N$13
  Top 0.3: U4.4 6.9,23.2 R8.2
N$14
  Top 0.3: R8.1 3.01,23.2 LED2.A
N$15
  Top 0.2: C28.2 R17.2 R16.2
N$16
  Top 0.3: R20.1 36.3,29.32 36.3,28.2 35.8,27.7 34.14,27.7 33.44,27 U1.47
N$17  (via drill 0.35)
  Top 0.2: v41.3,18.46 41.3,18.4 40.84,18.86 U1.25 | JP12.1 46.88,9.35 R4.1 45.3,12.5 44.4,13.4 v44.4,15.9
  Bottom 0.2: v44.4,15.9 41.84,18.46 v41.3,18.46
N$20
  Top 0.2: R3.2 27.54,22.86 28.81,21.59 29.94,20.46 30.04,20.36 U1.9
RESET  (via drill 0.3)
  Top 0.152: SW1.3 SW1.4
  Top 0.2: C19.1 R2.1 34.8,32.38 R30.1 34.59,31.33 U3.3 | SW1.3 3.34,47.53 3.81,48.01 | 11.09,48.01 SW1.4 20.17,47.53 20.97,46.73 20.97,46.3 22.2,45.07 22.2,41.67 v22.13,41.6 | C19.1 34.72,34.08 34.98,34.08 35.9,35 38.61,35 43.11,30.5 v44.4,30.5 | v57.5,24.9 56.97,24.9 52.57,29.3 v48.8,29.3 | C19.1 33.64,34.04 v33.6,34
  Bottom 0.2: v22.13,41.6 23.03,40.7 33.1,40.7 33.6,40.2 v33.6,34 | JP1.5 63.13,24.9 v57.5,24.9 57.5,22.93 43.66,9.09 42.1,9.09 38.26,5.25 35.73,5.25 U$4.RESET | v44.4,30.5 45.6,29.3 v48.8,29.3
RESET_W
  Top 0.2: R30.2 33.42,29.34 33.26,29.18 U3.2 32.94,28.86 U1.48
RXIN
  Top 0.2: P3.6 17.75,35.36 R17.1 20.75,32.36 20.75,31.25 21.17,30.83 22.39,30.83 23.03,30.18 23.03,27.29 23.89,26.43 26.84,26.43 28.23,25.04 28.23,23.93 29.8,22.36 U1.5
RXIP
  Top 0.2: 19.86,31.7 19.86,31.14 20.5,30.5 22.25,30.5 22.7,30.05 22.7,26.95 23.55,26.1 26.7,26.1 27.9,24.9 27.9,23.8 29.84,21.86 U1.6 | 19.86,31.7 R16.1 | 19.86,31.7 19.11,32.45 17.97,32.45 17.13,32.45 P3.3
SCK3
  Top 0.2: U6.4 50.36,14.84 52.11,13.09 P2.5
SCL
  Top 0.2: 18.95,50.05 21.3,47.7 21.3,46.5 23.35,44.45 JP3.4 | 18.95,50.05 18.8,50.2 | U$4.SCL 18.8,50.2 | 18.8,50.2 18.95,50.05
  Bottom 0.2: JP3.4 JP2.4
SCLK  (via drill 0.3, 0.35)
  Top 0.2: v42,21.07 41.95,21.12 41.16,21.12 40.91,21.36 U1.30 | U6.2 46.41,15.49 45.6,16.3 v45.6,18.82 | v57.7,26.7 56.51,27.89 55.95,27.89 55.53,28.32 v55.32,28.32 | v47.47,33.43 47.14,33.1 R23.2
  Bottom 0.2: JP1.3 58.94,27.94 v57.7,26.7 | v42,21.07 43.17,21.07 45.42,18.82 v45.6,18.82 45.85,19.07 46.13,19.07 46.41,19.35 49.37,19.35 56.66,26.64 57.64,26.64 v57.7,26.7 | 57.91,26.91 v57.7,26.7 | v55.32,28.32 50.2,33.43 v47.47,33.43
SDA
  Top 0.2: JP3.3 25.88,43.66 25.88,44.86 24.94,45.8 22.53,45.8 21.63,46.7 21.63,50.51 U$4.SDA
  Bottom 0.2: JP3.3 JP2.3
SEN3
  Top 0.2: U7.4 51.48,19.42 52.2,18.7 52.2,16.7 52.51,16.39 P2.2
SPD_N
  Top 0.2: LED4.K 48.71,31.5 43.62,26.4 43.62,17.08 41.15,14.62 36.99,14.62 35.44,16.18 U1.18
TXON  (via drill 0.3)
  Top 0.2: v24.5,29.5 26.71,29.5 29.58,26.64 29.58,24.59 30.3,23.86 30.4,23.86 31.24,23.86 31.25,23.86 U1.2 | R15.1 19.23,30.13 19.23,30.14 17.93,31.43 P3.2
  Bottom 0.2: v24.5,29.5 24.45,29.5 24.08,29.13 20.23,29.13 R15.1
  other vias: 19.86,29.5
TXOP  (via drill 0.3)
  Top 0.2: v24.5,28.67 27.08,28.67 29.25,26.5 29.25,24.45 30.34,23.36 U1.3 | R14.1 19.6,28 18.9,28.7 18.9,30 18.48,30.43 P3.1
  Bottom 0.2: v24.5,28.67 24.37,28.8 20.66,28.8 R14.1
  other vias: 19.86,28
XSCI
  Top 0.2: C1.2 27.05,17.35 Y1.3 28.49,17.44 R1.1 28.7,17.9 29.66,18.86 U1.12
XSCO
  Top 0.2: 28.77,19.36 R1.2 28.56,19.29 | 28.56,19.29 27.77,18.5 26.2,18.5 25.36,19.34 Y1.1 25.36,21.25 C2.2 | U1.11 28.64,19.36 28.56,19.29

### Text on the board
tNames: JP11 | JP10 | JP12 | Y1 | JP8 | JP9
tSILK: RESET | SCL | SDA | AREG | GND | 13 | 12 | 11 | 10 | 9 | 8 | 7 | 6 | 5 | 4 | 3 | 2 | 1 | 0 | OUT6 | OUT5 | IN2 | IN3 | COLn | TWI | TWI | ACTn | DPXn | SPDn | LINKn | 37 | W5100S Ethernet Shield | 1 | L | ON | 25 | 13 | IOREF | RESET | 3.3V | 5V | GND | GND | Vin | A0 | A1 | A2 | A3 | A4 | A5
bSILK: TX | RX | W5100S Ethernet Shield | OPEN-SOURCE ELECTRONICS | PROTOTYPING PLATFORM | http://wiznet.io | MADE IN KOREA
